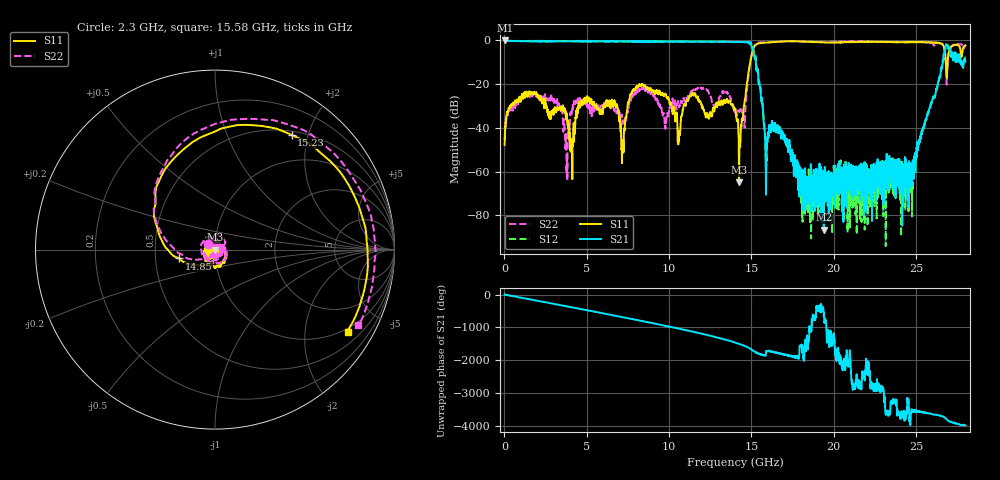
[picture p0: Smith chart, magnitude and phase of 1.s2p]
! 4/12/2023 4:31:05 PM
! D:\_XLC\ZLPF1-M0-15G-006\1.S2P
! CHANNEL.1
! TR.MEASUREMENT
! CORRECTED.DATA
! RF.CORRECTION: FULL.TWO.PORT.CAL.PORT.1.2
! AVERAGING.OFF
! IF.BANDWIDTH: 100KHZ
! SWEEPTYPE:  FREQ.SWEEP(Linear)
! Reference Plane Port Info
! PORT:  PORT1  PORT2
! DISTANCE:  0  m  0  m
! TIME:  0  s  0  s
! PHASE.OFFSET:  0 °  0 °
! LOSS:  0  dB  0  dB
! REF.LOSS:  0  dB  0  dB
! REF.FREQ:  0  Hz  0  Hz
! Power Info
! POWER:  -10  dBm  -10  dBm
! EFF.POWER:  -10  dBm  -10  dBm
! SOURCE.ATTEN:  0  dB  0  dB
! TEST.ATTEN:  0  dB  0  dB
# GHZ S RI R 50.0
! FREQ.GHZ  S11RE  S11IM  S21RE  S21IM  S12RE  S12IM  S22RE  S22IM
!; PortSelection: Port_12
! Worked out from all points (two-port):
!   2800 points, 10 MHz to 28 GHz, reference 50 ohm
!   highest |S21| = -0.04 dB at 20 MHz (marker M1); lowest = -86.5 dB at 19.4 GHz (marker M2)
!   |S21| within 3 dB of the highest: start of sweep to 15.01 GHz; 26.79 GHz to 26.93 GHz (141.1 MHz wide, 0.525 % of centre)
!   lowest |S11| = -64.8 dB at 14.25 GHz (marker M3), VSWR 1.00, Z = 50 - j0.0363 ohm
!   |S11| at or under -10 dB: start of sweep to 14.93 GHz; 26.81251 GHz to 26.91875 GHz (106.2 MHz wide, 0.395 % of centre)
!   |S22| runs from -64.1 to -0.3 dB; largest |S21 - S12| = 0.23
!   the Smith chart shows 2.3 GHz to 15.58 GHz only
!   S11 on the Smith chart (normalised r, x): 2.3 GHz: 0.93, +0.00; 14.85 GHz: 0.66, -0.07; 15.23 GHz: 0.55, +1.73; 15.58 GHz: 0.87, -3.30
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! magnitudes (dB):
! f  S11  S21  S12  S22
! 10 MHz  -47.8  0.0  0.0  -45.4
! 20 MHz  -44.9  0.0  0.0  -45.1
! 2.3 GHz  -28.2  -0.5  -0.4  -26.5
! 3.81 GHz  -36.9  -0.4  -0.3  -55.8
! 4.68 GHz  -28.5  -0.5  -0.4  -27.8
! 7.17 GHz  -45.8  -0.5  -0.4  -38.1
! 7.77 GHz  -23.3  -0.4  -0.3  -25.2
! 9.34 GHz  -24.4  -0.6  -0.5  -28.6
! 10.62 GHz  -41.5  -0.5  -0.5  -29.8
! 11.46 GHz  -24.8  -0.5  -0.6  -22.7
! 14.01 GHz  -31.5  -0.7  -0.7  -32.0
! 14.25 GHz  -64.8  -0.7  -0.7  -32.5
! 14.85 GHz  -13.7  -1.3  -0.7  -14.5
! 15.23 GHz  -2.3  -7.7  -8.5  -1.9
! 15.58 GHz  -1.2  -26.0  -25.2  -0.9
! 15.92 GHz  -1.0  -53.0  -56.0  -0.9
! 18.67 GHz  -0.7  -67.5  -70.5  -0.7
! 19.4 GHz  -1.0  -86.5  -76.3  -0.7
! 23.34 GHz  -0.7  -54.4  -69.6  -0.7
! 24.66 GHz  -0.8  -67.2  -60.5  -0.8
! 26.84 GHz  -14.1  -1.9  -2.3  -15.3
! 28 GHz  -2.3  -9.6  -7.8  -2.5
